| TEXAS INSTRUMENTS INCORPORATED
| Standard Linear and Logic Group
| IBIS Model of SN74LVCH16240A
| 16-Bit Buffer/Driver With 3-State Outputs
| This file contains package information for the following:
|  TSSOP 48-pin (DGG) package as [Component] LVCH16240_DGG
|  SSOP 48-pin (DL) package as [Component] LVCH16240_DL
| This device can be powered at the following Vccs:
|  3.3 volt Vcc
|  2.5 volt Vcc
|  1.8 volt Vcc
| This file provides unique models under the [Model Selector] for each Vcc.
| For operation at a specific Vcc, select the appropriate model after each
| [Model Selector] keyword.
[IBIS Ver]   3.2
[Comment char]  |_char
[File Name]   sn74lvch16240a.ibs
[File Rev]   1.1 | e_die
[Date]   March 1, 2001
[Source]   Data created from TI-SPICE simulations at TI-SLL.
[Notes]   The following is an IBIS list for the LVCH16240.
   Please contact sllibis@ti.com with questions and
   comments concerning SLL IBIS models.
		Power clamp data deleted as there is no power-clamp diode.
		Non monotonic warning in ground clamp due to bus-hold.
		C_comp values are taken at a different test condition
		than the data sheet.
[Disclaimer] Property of Texas Instruments Incorporated.  Unauthorized
   reproduction and/or distribution is strictly prohibited.
   This product is protected under copyright law.
   Created  2001, (C) Copyright  2001, Texas Instruments
   Incorporated, All Rights Reserved
   UNLESS THERE IS A SIGNED, WRITTEN AGREEMENT TO THE
   CONTRARY, TEXAS INSTRUMENTS (TI) IS PROVIDING THE IBIS
   MODELS  AND WITHOUT ANY WARRANTY, EXPRESSED OR
   IMPLIED.  TI assumes no liability for:
   1) the accuracy of the IBIS models provided to your
   company;
   2) the proper functioning of these IBIS Models in your
   design or for any resulting applications; or
   3) infringement of patents, copyrights or intellectual
   property rights resulting from your use of these IBIS
   models.
   TI provides IBIS Models as a service to our customers.
   You and your company shall not distribute, sell or give
   these models to anyone else without prior written
   permission from TI.
   TI reserves the right to make changes to our products or
   to discontinue any semiconductor product or service
   without notice, and advises our customers to obtain the
   latest version of relevant information to verify, before
   placing orders, that the information being relied on is
   current.
   Please be aware that your receipt and use of the IBIS
   information provided shall serve as acceptance of these
   terms and conditions.  If you do not accept these terms,
   you should return or destroy the IBIS models and any
   other accompanying information immediately.
| Component LVCH16240_DGG 48-pin TSSOP
[Component]   LVCH16240_DGG
[Manufacturer]   Texas Instruments, Inc.
[Package]
|   typ   min   max
R_pkg   6.200e-02   5.000e-02   7.800e-02
L_pkg   3.527e-09   3.128e-09   4.255e-09
C_pkg   5.300e-13   4.170e-13   6.850e-13
[Pin]   signal_name   model_name   R_pin   L_pin   C_pin
1   1OE   LVCH16240_OEIN   5.000e-02   4.250e-09   6.710e-13
2   1Y1   LVCH16240_OUT   5.700e-02   3.956e-09   6.740e-13
3   1Y2   LVCH16240_OUT   7.100e-02   3.922e-09   6.190e-13
4   GND   GND   7.800e-02   3.841e-09   6.180e-13
5   1Y3   LVCH16240_OUT   5.600e-02   3.535e-09   5.550e-13
6   1Y4   LVCH16240_OUT   5.800e-02   3.464e-09   5.030e-13
7   VCC   POWER   6.000e-02   3.362e-09   4.980e-13
8   2Y1   LVCH16240_OUT   6.100e-02   3.293e-09   4.620e-13
9   2Y2   LVCH16240_OUT   6.300e-02   3.240e-09   4.550e-13
10   GND   GND   6.300e-02   3.175e-09   4.420e-13
11   2Y3   LVCH16240_OUT   6.400e-02   3.153e-09   4.290e-13
12   2Y4   LVCH16240_OUT   6.500e-02   3.128e-09   4.180e-13
13   3Y1   LVCH16240_OUT   6.500e-02   3.128e-09   4.180e-13
14   3Y2   LVCH16240_OUT   6.400e-02   3.154e-09   4.290e-13
15   GND   GND   6.300e-02   3.174e-09   4.420e-13
16   3Y3   LVCH16240_OUT   6.300e-02   3.241e-09   4.550e-13
17   3Y4   LVCH16240_OUT   6.100e-02   3.293e-09   4.620e-13
18   VCC   POWER   6.000e-02   3.362e-09   4.970e-13
19   4Y1   LVCH16240_OUT   5.800e-02   3.464e-09   5.030e-13
20   4Y2   LVCH16240_OUT   5.600e-02   3.537e-09   5.600e-13
21   GND   GND   7.700e-02   3.839e-09   6.260e-13
22   4Y3   LVCH16240_OUT   7.100e-02   3.917e-09   6.270e-13
23   4Y4   LVCH16240_OUT   5.800e-02   3.955e-09   6.850e-13
24   4OE   LVCH16240_OEIN   5.200e-02   4.255e-09   6.790e-13
25   3OE   LVCH16240_OEIN   5.100e-02   4.254e-09   6.760e-13
26   4A4   LVCH16240_IN   5.800e-02   3.957e-09   6.790e-13
27   4A3   LVCH16240_IN   7.100e-02   3.920e-09   6.210e-13
28   GND   GND   7.800e-02   3.843e-09   6.220e-13
29   4A2   LVCH16240_IN   5.600e-02   3.539e-09   5.600e-13
30   4A1   LVCH16240_IN   5.800e-02   3.466e-09   5.030e-13
31   VCC   POWER   6.000e-02   3.363e-09   4.970e-13
32   3A4   LVCH16240_IN   6.100e-02   3.294e-09   4.620e-13
33   3A3   LVCH16240_IN   6.300e-02   3.241e-09   4.540e-13
34   GND   GND   6.300e-02   3.175e-09   4.410e-13
35   3A2   LVCH16240_IN   6.400e-02   3.153e-09   4.290e-13
36   3A1   LVCH16240_IN   6.500e-02   3.129e-09   4.170e-13
37   2A4   LVCH16240_IN   6.500e-02   3.129e-09   4.170e-13
38   2A3   LVCH16240_IN   6.400e-02   3.152e-09   4.290e-13
39   GND   GND   6.400e-02   3.176e-09   4.410e-13
40   2A2   LVCH16240_IN   6.300e-02   3.241e-09   4.540e-13
41   2A1   LVCH16240_IN   6.100e-02   3.293e-09   4.620e-13
42   VCC   POWER   6.000e-02   3.363e-09   4.970e-13
43   1A4   LVCH16240_IN   5.800e-02   3.464e-09   5.030e-13
44   1A3   LVCH16240_IN   5.600e-02   3.534e-09   5.610e-13
45   GND   GND   7.800e-02   3.841e-09   6.260e-13
46   1A2   LVCH16240_IN   7.100e-02   3.920e-09   6.220e-13
47   1A1   LVCH16240_IN   5.700e-02   3.955e-09   6.770e-13
48   2OE   LVCH16240_OEIN   5.100e-02   4.252e-09   6.720e-13
| Component LVCH16240_DL 48-pin SSOP
[Component]   LVCH16240_DL
[Manufacturer]   Texas Instruments, Inc.
[Package]
|   typ   min   max
R_pkg   4.800e-02   3.800e-02   5.300e-02
L_pkg   6.046e-09   5.084e-09   7.968e-09
C_pkg   8.130e-13   5.690e-13   1.157e-12
[Pin]   signal_name   model_name   R_pin   L_pin   C_pin
1   1OE   LVCH16240_OEIN   4.600e-02   7.968e-09   1.017e-12
2   1Y1   LVCH16240_OUT   4.400e-02   7.299e-09   1.157e-12
3   1Y2   LVCH16240_OUT   4.300e-02   6.765e-09   1.058e-12
4   GND   GND   4.100e-02   6.269e-09   9.330e-13
5   1Y3   LVCH16240_OUT   3.800e-02   5.856e-09   8.290e-13
6   1Y4   LVCH16240_OUT   4.600e-02   5.802e-09   7.900e-13
7   VCC   POWER   5.000e-02   5.656e-09   7.380e-13
8   2Y1   LVCH16240_OUT   5.300e-02   5.500e-09   6.430e-13
9   2Y2   LVCH16240_OUT   5.200e-02   5.304e-09   6.060e-13
10   GND   GND   5.300e-02   5.189e-09   5.830e-13
11   2Y3   LVCH16240_OUT   5.100e-02   5.084e-09   5.690e-13
12   2Y4   LVCH16240_OUT   5.300e-02   5.862e-09   8.330e-13
13   3Y1   LVCH16240_OUT   5.300e-02   5.862e-09   8.330e-13
14   3Y2   LVCH16240_OUT   5.100e-02   5.084e-09   5.690e-13
15   GND   GND   5.300e-02   5.189e-09   5.830e-13
16   3Y3   LVCH16240_OUT   5.200e-02   5.304e-09   6.060e-13
17   3Y4   LVCH16240_OUT   5.300e-02   5.500e-09   6.430e-13
18   VCC   POWER   5.000e-02   5.656e-09   7.380e-13
19   4Y1   LVCH16240_OUT   4.600e-02   5.802e-09   7.900e-13
20   4Y2   LVCH16240_OUT   3.800e-02   5.856e-09   8.290e-13
21   GND   GND   4.100e-02   6.269e-09   9.330e-13
22   4Y3   LVCH16240_OUT   4.300e-02   6.765e-09   1.058e-12
23   4Y4   LVCH16240_OUT   4.400e-02   7.299e-09   1.157e-12
24   4OE   LVCH16240_OEIN   4.600e-02   7.968e-09   1.017e-12
25   3OE   LVCH16240_OEIN   4.600e-02   7.968e-09   1.017e-12
26   4A4   LVCH16240_IN   4.400e-02   7.299e-09   1.157e-12
27   4A3   LVCH16240_IN   4.300e-02   6.765e-09   1.058e-12
28   GND   GND   4.100e-02   6.269e-09   9.330e-13
29   4A2   LVCH16240_IN   3.800e-02   5.856e-09   8.290e-13
30   4A1   LVCH16240_IN   4.600e-02   5.802e-09   7.900e-13
31   VCC   POWER   5.000e-02   5.656e-09   7.380e-13
32   3A4   LVCH16240_IN   5.300e-02   5.500e-09   6.430e-13
33   3A3   LVCH16240_IN   5.200e-02   5.304e-09   6.060e-13
34   GND   GND   5.300e-02   5.189e-09   5.830e-13
35   3A2   LVCH16240_IN   5.100e-02   5.084e-09   5.690e-13
36   3A1   LVCH16240_IN   5.300e-02   5.862e-09   8.330e-13
37   2A4   LVCH16240_IN   5.300e-02   5.862e-09   8.330e-13
38   2A3   LVCH16240_IN   5.100e-02   5.084e-09   5.690e-13
39   GND   GND   5.300e-02   5.189e-09   5.830e-13
40   2A2   LVCH16240_IN   5.200e-02   5.304e-09   6.060e-13
41   2A1   LVCH16240_IN   5.300e-02   5.500e-09   6.430e-13
42   VCC   POWER   5.000e-02   5.656e-09   7.380e-13
43   1A4   LVCH16240_IN   4.600e-02   5.802e-09   7.900e-13
44   1A3   LVCH16240_IN   3.800e-02   5.856e-09   8.290e-13
45   GND   GND   4.100e-02   6.269e-09   9.330e-13
46   1A2   LVCH16240_IN   4.300e-02   6.765e-09   1.058e-12
47   1A1   LVCH16240_IN   4.400e-02   7.299e-09   1.157e-12
48   2OE   LVCH16240_OEIN   4.600e-02   7.967e-09   1.017e-12
| Model LVCH16240_OEIN
[Model Selector]   LVCH16240_OEIN
LVCH16240_OEIN_33   3.3 volt Vcc
LVCH16240_OEIN_25   2.5 volt Vcc
LVCH16240_OEIN_18   1.8 volt Vcc
| Model LVCH16240_IN
[Model Selector]   LVCH16240_IN
LVCH16240_IN_33   3.3 volt Vcc
LVCH16240_IN_25   2.5 volt Vcc
LVCH16240_IN_18   1.8 volt Vcc
| Model LVCH16240_OUT
[Model Selector]   LVCH16240_OUT
LVCH16240_OUT_33   3.3 volt Vcc
LVCH16240_OUT_25   2.5 volt Vcc
LVCH16240_OUT_18   1.8 volt Vcc
| Models and submodels in the file (9): LVCH16240_OEIN_33 (Input), LVCH16240_OEIN_25 (Input), LVCH16240_OEIN_18 (Input), LVCH16240_IN_33 (Input), LVCH16240_IN_25 (Input), LVCH16240_IN_18 (Input), LVCH16240_OUT_33 (3-state), LVCH16240_OUT_25 (3-state), LVCH16240_OUT_18 (3-state)
